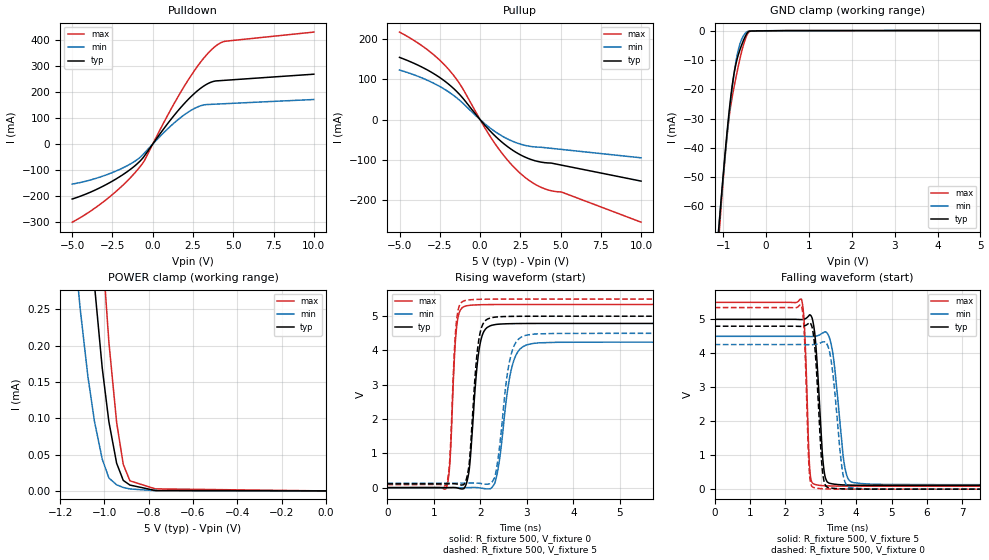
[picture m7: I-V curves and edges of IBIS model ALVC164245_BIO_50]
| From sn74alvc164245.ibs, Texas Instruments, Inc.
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[Model]   ALVC164245_BIO_50
Model_type  I/O
Vinl = 0.8
Vinh = 2
Enable   Active-Low
Vref =   0
Rref =   500
Cref =   50p
Vmeas =   1.5
| variable   typ   min   max
C_comp   8.5pF   NA   NA
| C_pullup   3.13pF   2.71pF   3.71pF
| C_pulldown   3.89pF   2.65pF   5.54pF
| C_tri-state   2.69pF   2.30pF   3.44pF
[Temperature Range]   40   100   -40
| Ambient temperature   25   85   -40
[Voltage range]   5   4.5   5.5
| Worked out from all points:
|   slope of the pulldown table from 0 to 0.75 V, typ, clamps not added: 11.7 ohm
|   slope of the pullup table from 0 to 0.75 V, typ, clamps not added: 22.5 ohm
|   GND clamp passes 1 mA (typ) near -0.45 V on its own axis
|   POWER clamp passes 1 mA (typ) near -1.18 V on its own axis
|   rising waveform, R_fixture 500, V_fixture 0: 20-80 % time 163ps typ, 242ps min, 105ps max; typ from 0 V to 4.79 V
|   falling waveform, R_fixture 500, V_fixture 5: 20-80 % time 166ps typ, 243ps min, 105ps max; typ from 5 V to 0.111 V
|   rising waveform, R_fixture 500, V_fixture 5: 20-80 % time 154ps typ, 224ps min, 104ps max; typ from 0.111 V to 5 V
|   falling waveform, R_fixture 500, V_fixture 0: 20-80 % time 157ps typ, 232ps min, 101ps max; typ from 4.8 V to 0 V
[GND Clamp]
| ALVC164245_BIO_50
|   Voltage   I(typ)   I(min)   I(max)
-5V       -865.1mA   -810.7mA   -942.2mA
-1.11V    -68.65mA   -68.11mA   -72.05mA
-1.09V    -64.99mA   -64.68mA   -68.03mA
-1.07V    -61.37mA   -61.28mA   -64.08mA
-970mV    -44.01mA   -44.85mA   -45.45mA
-890mV    -31.43mA   -32.66mA   -33.03mA
-770mV    -16.63mA   -17.04mA   -20.93mA
-700mV    -11.11mA   -10.21mA   -15.72mA
-620mV    -6.918mA   -4.99mA    -10.18mA
-435mV    -692uA     -275.7uA   -1.167mA
-180mV    -68.49uA   -47.87uA   -99.9uA
5V        9.439uA    66.99uA    116.8uA
[POWER Clamp]
| ALVC164245_BIO_50
|   Voltage   I(typ)   I(min)   I(max)
-5V       112.4mA    87.95mA    157.3mA
-1.14V    741.3uA    349.9uA    1.269mA
-1.11V    574uA      252.1uA    1.003mA
-1.075V   405.2uA    158.3uA    730.2uA
-1.045V   283.6uA    95.72uA    529.9uA
-1.01V    169.2uA    43.84uA    336.1uA
-980mV    95.42uA    17.87uA    205.1uA
-945mV    38.19uA    8.406uA    94.4uA
-915mV    14.48uA    4.781uA    36.58uA
-885mV    8.065uA    2.727uA    13.9uA
-770mV    544.7nA    327.6nA    2.839uA
-84.45fV  66pA       1.406nA    401.9pA
[Pulldown]
| ALVC164245_BIO_50
|   Voltage   I(typ)   I(min)   I(max)
-5V       -211.2mA   -153.8mA   -300.3mA
-3.875V   -185.1mA   -138.2mA   -258.2mA
-2.735V   -150.4mA   -115mA     -205.8mA
-1.675V   -110.1mA   -86.17mA   -147.5mA
-855mV    -69.45mA   -54.64mA   -91.96mA
-510mV    -45.04mA   -33.83mA   -62.59mA
895mV     76.14mA    56.51mA    107mA
2.02V     159.6mA    115.1mA    228.4mA
3.06V     218.3mA    148.5mA    321.8mA
3.895V    242.2mA    153.3mA    375.9mA
4.525V    245mA      155.2mA    395.3mA
10V       268.3mA    171.1mA    430.2mA
[Pullup]
| ALVC164245_BIO_50
|   Voltage   I(typ)   I(min)   I(max)
-5V       153.7mA    122.5mA    216.2mA
-3.255V   122.3mA    96.93mA    172.2mA
-2.535V   104.8mA    82.57mA    148mA
-1.905V   85.97mA    67.15mA    122mA
-1.135V   56.04mA    42.98mA    80.39mA
235mV     -11.1mA    -8.276mA   -16.21mA
1.03V     -44.16mA   -32.3mA    -65.34mA
1.925V    -73.11mA   -52.05mA   -110.1mA
2.82V     -93.3mA    -64.07mA   -143.7mA
3.97V     -106.4mA   -69.3mA    -170.6mA
5.04V     -112.6mA   -73.78mA   -179mA
10V       -152.2mA   -94.6mA    -253.8mA
[Ramp]
| ALVC164245_BIO_50
| variable   typ   min   max
dV/dt_r   2.90/1.69E-10   2.57/2.46E-10   3.23/1.08E-10
dV/dt_f   3.01/1.77E-10   2.70/2.59E-10   3.31/1.09E-10
R_load = 500
[Rising Waveform]
| ALVC164245_BIO_50
R_fixture =   500
C_fixture =   0
L_fixture =   0
V_fixture =   0
V_fixture_min = 0
V_fixture_max = 0
|   Time   V(typ)   V(min)   V(max)
0s        125.9pV    3.401nV    33.85nV
1.265ns   -47.32uV   26.68uV    -25.91mV
1.345ns   1.252mV    -13.92uV   743.2mV
1.5ns     -7.23mV    -147.4uV   4.797V
1.81ns    1.324V     3.687mV    5.322V
2.08ns    4.565V     -26.48mV   5.337V
2.345ns   4.761V     299.5mV    5.341V
2.735ns   4.784V     3.764V     5.342V
3.265ns   4.789V     4.223V     5.342V
50ns      4.789V     4.244V     5.342V
[Falling Waveform]
| ALVC164245_BIO_50
R_fixture =   500
C_fixture =   0
L_fixture =   0
V_fixture =   5
V_fixture_min = 4.5
V_fixture_max = 5.5
|   Time   V(typ)   V(min)   V(max)
0s        5V         4.5V       5.5V
2.45ns    4.993V     4.5V       5.597V
2.54ns    5.01V      4.498V     4.719V
2.7ns     5.128V     4.494V     439.2mV
2.835ns   4.513V     4.502V     140.5mV
2.99ns    1.998V     4.558V     109.7mV
3.17ns    228.2mV    4.603V     97.89mV
3.7ns     122.9mV    532.9mV    89.34mV
4.145ns   114.5mV    165.5mV    88.19mV
50ns      110.5mV    131.6mV    87.73mV
[Rising Waveform]
| ALVC164245_BIO_50
R_fixture =   500
C_fixture =   0
L_fixture =   0
V_fixture =   5
V_fixture_min = 4.5
V_fixture_max = 5.5
|   Time   V(typ)   V(min)   V(max)
0s        110.5mV    131.6mV    87.73mV
1.265ns   110.5mV    131.6mV    66.79mV
1.34ns    111.6mV    131.6mV    771.8mV
1.5ns     103.3mV    131.4mV    5.006V
1.785ns   1.097V     134.1mV    5.479V
2.055ns   4.77V      111.6mV    5.495V
2.325ns   4.974V     384.5mV    5.499V
2.695ns   4.995V     4.032V     5.5V
3.19ns    4.999V     4.482V     5.5V
50ns      5V         4.5V       5.5V
[Falling Waveform]
| ALVC164245_BIO_50
R_fixture =   500
C_fixture =   0
L_fixture =   0
V_fixture =   0
V_fixture_min = 0
V_fixture_max = 0
|   Time   V(typ)   V(min)   V(max)
0s        4.798V     4.258V     5.346V
2.45ns    4.792V     4.258V     5.416V
2.535ns   4.807V     4.256V     4.511V
2.685ns   4.907V     4.253V     370.3mV
2.945ns   2.23V      4.287V     19.61mV
3.115ns   147.1mV    4.338V     8.742mV
3.31ns    30.61mV    3.644V     4.049mV
3.635ns   8.53mV     386.2mV    1.261mV
3.995ns   3.009mV    27.69mV    416.2uV
50ns      4.405uV    7.174uV    4.139uV
